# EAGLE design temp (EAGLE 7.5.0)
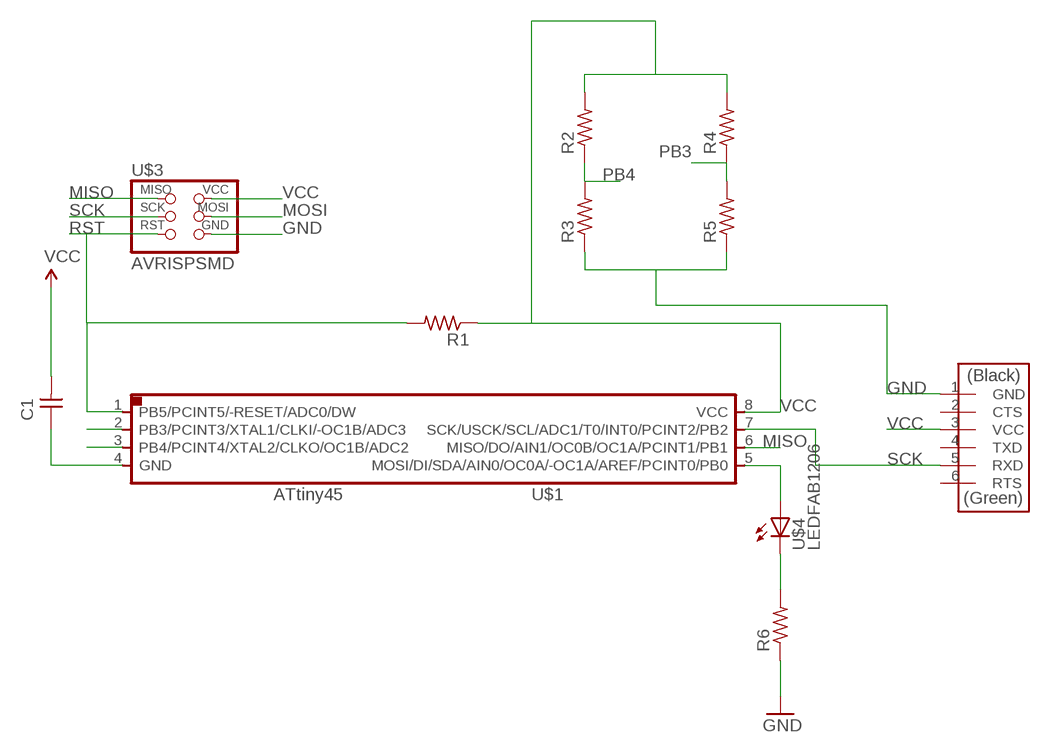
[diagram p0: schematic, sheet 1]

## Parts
C1  CAP-UNPOLARIZEDFAB  [C1206FAB]
R1  RES-US1206FAB  [R1206FAB]
R2  RES-US1206FAB  [R1206FAB]
R3  RES-US1206FAB  [R1206FAB]
R4  RES-US1206FAB  [R1206FAB]
R5  RES-US1206FAB  [R1206FAB]
R6  RES-US1206FAB  [R1206FAB]
U$1  Tiny45  ATTINY45SI  [SOIC8]
U$2  FTDI-SMD-HEADER  [1X06SMD]
U$3  AVRISPSMD  [2X03SMD]
U$4  LEDFAB1206  [LED1206FAB]

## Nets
GND: C1.1 R3.1 R5.1 R6.1 U$1.4(GND) U$2.1(GND) U$3.6(GND)
MISO: U$1.6(MISO/DO/AIN1/OC0B/OC1A/PCINT1/PB1) U$3.1(MISO)
MOSI: U$1.5(MOSI/DI/SDA/AIN0/OC0A/-OC1A/AREF/PCINT0/PB0) U$3.4(MOSI) U$4.1(A)
N$1: R6.2 U$4.2(C)
PB3: R4.1 R5.2 U$1.2(PB3/PCINT3/XTAL1/CLKI/-OC1B/ADC3)
PB4: R2.1 R3.2 U$1.3(PB4/PCINT4/XTAL2/CLKO/OC1B/ADC2)
RST: R1.2 U$1.1(PB5/PCINT5/-RESET/ADC0/DW) U$3.5(RST)
SCK: U$1.7(SCK/USCK/SCL/ADC1/T0/INT0/PCINT2/PB2) U$2.5(RXD) U$3.3(SCK)
VCC: C1.2 R1.1 R2.2 R4.2 U$1.8(VCC) U$2.3(VCC) U$3.2(VCC)
Unconnected: U$2.2(CTS) U$2.4(TXD) U$2.6(RTS)

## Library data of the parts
C1 = fab:CAP-UNPOLARIZED
R1-R6 = fab:RES-US: Resistor (US Symbol)
U$1 = fab:ATTINY45
U$2 = fab:FTDI-SMD-HEADER
U$3 = fab:AVRISP
U$4 = fab:LED: LED

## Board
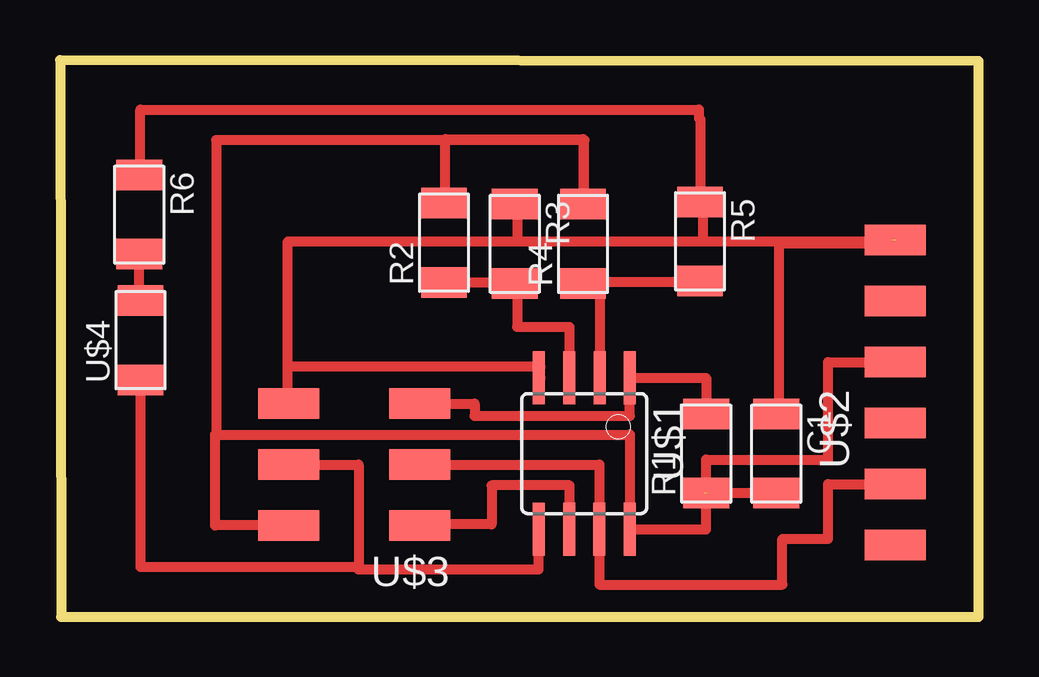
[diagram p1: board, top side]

Size 38.28 x 23.21 mm. Coordinates in mm from the lower left corner, seen from the top.
Outline: 0.05,0 38.28,0 38.28,23.15 0,23.21 0.05,0
Copper layers (1*16): Top 0.035mm / dielectric 1.5mm / Bottom 0.035mm
Design rules "default *": minimum track width 16mil, minimum drill 24mil, track to track 16mil, track to pad 16mil, pad to pad 8mil, via to via 8mil, smd to smd 8mil, copper to edge 40mil, drill to drill 8mil, minimum pad ring 10mil, minimum via ring 8mil, stop-mask expansion 4mil, vias tented up to drill 0mil, thermal gap 10mil

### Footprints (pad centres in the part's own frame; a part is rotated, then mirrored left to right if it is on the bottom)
C1206FAB = smd 1.27 x 1.905: 1 -1.651,0; 2 1.651,0
R1206FAB = smd 1.27 x 1.905: 1 -1.651,0; 2 1.651,0
SOIC8 = smd 0.5 x 2.2: 1 -1.905,-3.154; 2 -0.645,-3.154; 3 0.625,-3.154; 4 1.895,-3.154; 5 1.905,3.154; 6 0.635,3.154; 7 -0.635,3.154; 8 -1.905,3.154
1X06SMD = smd 2.54 x 1.27: 1 0,6.35; 2 0,3.81; 3 0,1.27; 4 0,-1.27; 5 0,-3.81; 6 0,-6.35
2X03SMD = smd 2.54 x 1.27: 1 -2.54,2.54; 2 2.92,2.54; 3 -2.54,0; 4 2.92,0; 5 -2.54,-2.54; 6 2.92,-2.54
LED1206FAB = smd 1.27 x 1.905: 1 -1.651,0; 2 1.651,0

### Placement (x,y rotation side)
C1  29.84,6.81 270 top
R1  26.92,6.81 90 top
R2  16,15.6 90 top
R3  18.95,15.54 270 top
R4  21.79,15.54 90 top
R5  26.67,15.65 270 top
R6  3.3,16.76 270 top
U$1  21.84,6.81 180 top
U$2  34.8,9.35 0 top
U$3  12.45,6.35 180 top
U$4  3.35,11.53 90 top

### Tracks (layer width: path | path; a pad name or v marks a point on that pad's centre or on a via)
GND  (1 unrouted)
  Top 0.406: U$3.6 9.5,9.09 9.5,10.41 | 9.5,10.41 9.5,15.65 19.05,15.65 | 19.05,15.65 26.77,15.65 | 26.77,15.65 34.8,15.65 U$2.1 | 26.77,15.65 26.77,17.3 R5.1 26.67,20.78 26.62,20.78 26.62,21.13 3.35,21.13 3.35,18.42 R6.1 | R3.1 19.05,17.2 19.05,15.65 | 34.67,15.7 34.67,15.57 29.97,15.57 29.97,8.46 C1.1 | U$1.4 20.02,9.96 20.02,10.41 9.5,10.41
MISO
  Top 0.406: 15.24,4.01 U$3.1 14.99,3.86 17.98,3.86 17.98,5.49 21.23,5.49 21.23,3.65 U$1.6
MOSI
  Top 0.406: U$1.5 19.94,1.98 12.45,1.98 12.45,2.08 | U$3.4 12.45,6.35 12.45,2.08 | 3.4,9.88 U$4.1 3.35,2.08 12.45,2.08
N$1
  Top 0.406: U$4.2 3.3,13.18 R6.2
PB3
  Top 0.406: R5.2 26.67,13.97 21.9,13.97 21.9,13.89 R4.1 22.49,13.89 U$1.2
PB4
  Top 0.406: 21.23,9.96 U$1.3 21.22,12.09 19.05,12.09 19.05,13.89 R3.2 18.95,13.94 R2.1
RST
  Top 0.406: R1.2 26.92,9.96 U$1.1 23.75,8.38 17.27,8.38 17.27,8.89 U$3.5
SCK
  Top 0.406: U$2.5 32,5.54 32,3.25 30.1,3.25 30.1,1.35 22.48,1.35 U$1.7 22.48,6.35 U$3.3
VCC  (1 unrouted)
  Top 0.406: U$2.3 32,10.62 32,6.55 26.92,6.55 R1.1 26.92,3.65 U$1.8 23.75,7.59 6.5,7.59 | R2.2 16.05,17.25 16.05,19.91 21.79,19.91 R4.2 21.84,17.2 21.84,19.86 6.5,19.86 6.5,7.59 | C1.2 26.87,5.16 26.87,5.08 | 6.5,7.59 6.45,7.59 6.45,3.81 U$3.2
